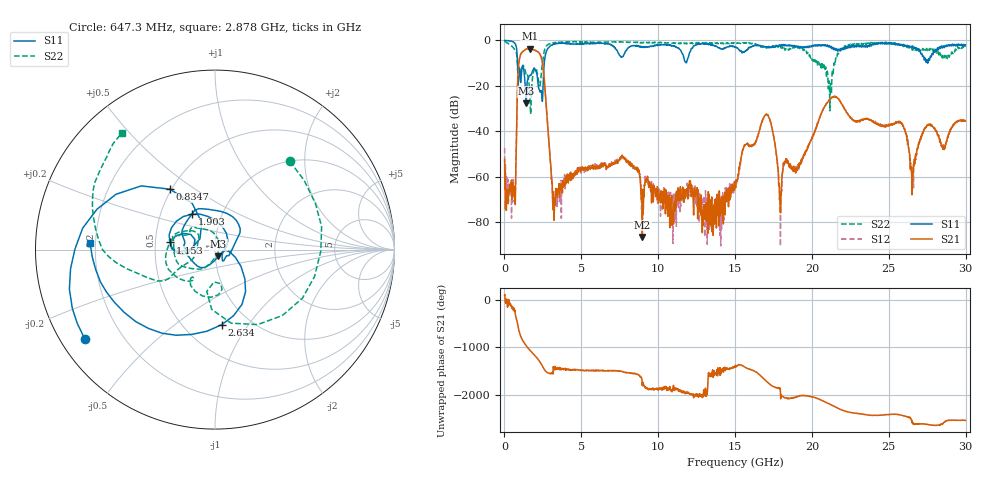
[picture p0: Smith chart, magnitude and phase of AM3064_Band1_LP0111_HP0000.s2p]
# Hz S DB R 50.0
!freq dBS11 angS11 dBS21 angS21 dBS12 angS12 dBS22 angS22
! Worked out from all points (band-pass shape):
!   1600 points, 10 MHz to 29.98 GHz, reference 50 ohm
!   highest |S21| = -3.64 dB at 1.641 GHz (marker M1); lowest = -86.6 dB at 8.97 GHz (marker M2)
!   |S21| within 3 dB of the highest: 1.03 GHz to 2.343 GHz (1.313 GHz wide, 77.8 % of centre)
!   lowest |S11| = -27.7 dB at 1.416 GHz (marker M3), VSWR 1.09, Z = 51.8 - j3.81 ohm
!   |S11| at or under -10 dB: 848.8 MHz to 2.588 GHz (1.739 GHz wide, 101 % of centre); 27.52473 GHz to 27.53172 GHz (6.986 MHz wide, 0.0254 % of centre)
!   |S22| runs from -32.5 to -0.3 dB; largest |S21 - S12| = 0.008
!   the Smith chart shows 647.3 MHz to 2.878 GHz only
!   S11 on the Smith chart (normalised r, x): 647.3 MHz: 0.07, -0.31; 834.7 MHz: 0.49, +0.40; 1.153 GHz: 0.60, +0.05; 1.903 GHz: 0.72, +0.30; 2.634 GHz: 0.75, -0.76; 2.878 GHz: 0.18, +0.02
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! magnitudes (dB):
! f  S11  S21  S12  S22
! 10 MHz  0.0  -52.5  -47.4  -0.3
! 647.3 MHz  -1.1  -66.6  -64.3  -3.8
! 834.7 MHz  -7.5  -24.6  -24.5  -9.5
! 1.153 GHz  -11.9  -5.2  -5.1  -11.7
! 1.416 GHz  -27.7  -3.8  -3.8  -15.3
! 1.641 GHz  -15.6  -3.6  -3.6  -23.0
! 1.903 GHz  -12.5  -4.1  -4.1  -13.2
! 2.634 GHz  -7.5  -21.1  -21.1  -3.7
! 2.878 GHz  -3.1  -43.7  -43.3  -1.6
! 3.271 GHz  -1.6  -69.3  -69.1  -0.9
! 5.015 GHz  -1.5  -56.0  -56.0  -0.7
! 8.97 GHz  -2.8  -86.6  -78.6  -1.0
! 10 GHz  -2.1  -65.8  -69.2  -0.9
! 15 GHz  -3.0  -62.0  -62.5  -1.4
! 16.99 GHz  -2.9  -32.7  -32.7  -3.1
! 17.95 GHz  -2.2  -76.0  -90.7  -2.8
! 19.99 GHz  -2.8  -43.1  -43.3  -8.1
! 21.42 GHz  -3.8  -24.8  -24.7  -11.1
! 25 GHz  -1.0  -37.4  -37.3  -1.1
! 26.53 GHz  -2.4  -63.2  -58.6  -4.3
! 27.45 GHz  -9.0  -38.1  -38.0  -3.5
! 29.98 GHz  -1.9  -35.5  -35.3  -2.8
